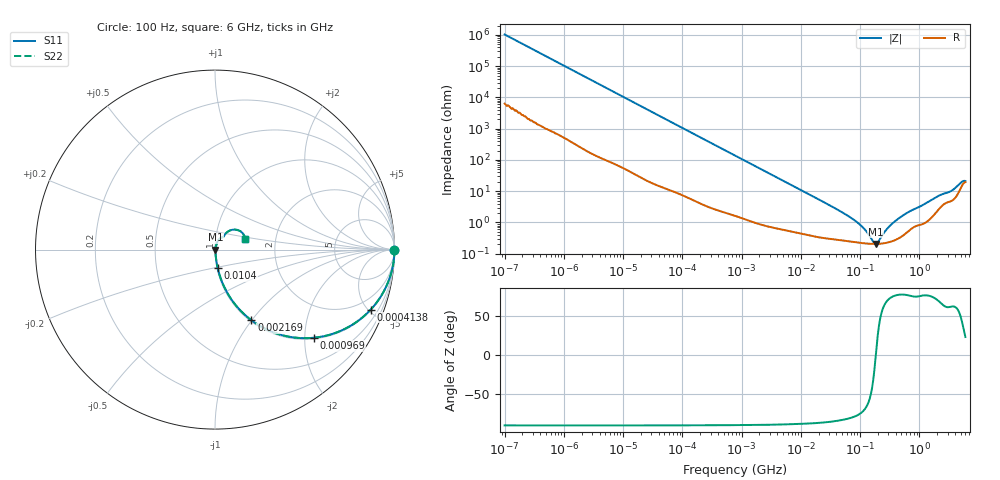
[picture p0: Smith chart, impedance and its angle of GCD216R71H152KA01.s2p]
!Murata Part Number: GCD216R71H152KA01
!These Parameters are Measured in Series Mode Connection
!Data Generated on Mar 13, 2026
!  o--ll--o
!Port1  Port2
!  o------o
!Operation Temp=25[degC], DC Bias Voltage=0[V]
!Freq. Start=100[Hz] Stop=6[GHz] 401[Steps]
# Hz S RI R 50
!Freq.(Hz) S11(Real) S11(Imag) S21(Real) S21(Imag) S12(Real) S12(Imag) S22(Real) S22(Imag)
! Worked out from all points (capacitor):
!   401 points, 100 Hz to 6 GHz, reference 50 ohm
!   read as one part in series: C = 1.53 nF near 109 Hz
!   lowest |Z| = 207 mohm at 182.6 MHz (marker M1)
!   series resonance near 184.5 MHz, so ESL is about 490 pH
!   S11 on the Smith chart (normalised r, x): 100 Hz: open; 413.8 kHz: 1.05, -5.16; 969 kHz: 1.03, -2.22; 2.169 MHz: 1.02, -0.99; 10.4 MHz: 1.01, -0.21; 6 GHz: 1.39, +0.17
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100  1 -9.63e-05  6e-07 9.63e-05  6e-07 9.63e-05  1 -9.63e-05
2008  1 -0.00192  1.24e-05 0.00192  1.24e-05 0.00192  1 -0.00192
40335  0.9983 -0.0381  0.00166 0.0381  0.00166 0.0381  0.9983 -0.0381
141303  0.9817 -0.1303  0.0183 0.1303  0.0183 0.1303  0.9817 -0.1303
413847  0.8672 -0.3348  0.1328 0.3348  0.1328 0.3348  0.8672 -0.3348
774597  0.6552 -0.4694  0.3448 0.4694  0.3448 0.4694  0.6552 -0.4694
968953  0.5504 -0.4911  0.4496 0.4911  0.4496 0.4911  0.5504 -0.4911
2169299  0.2025 -0.3934  0.7975 0.3934  0.7975 0.3934  0.2025 -0.3934
4060267  0.0716 -0.2463  0.9284 0.2463  0.9284 0.2463  0.0716 -0.2463
1.039699e7  0.0151 -0.1032  0.9849 0.1032  0.9849 0.1032  0.0151 -0.1032
1.555665e7  0.00854 -0.0696  0.9915 0.0696  0.9915 0.0696  0.00854 -0.0696
8.154455e7  0.00247 -0.0113  0.9975 0.0113  0.9975 0.0113  0.00247 -0.0113
1.166697e8  0.00219 -0.00597  0.9978 0.00597  0.9978 0.00597  0.00219 -0.00597
1.669249e8  0.00206 -0.00127  0.9979 0.00127  0.9979 0.00127  0.00206 -0.00127
1.825626e8  0.00206 -0.000133  0.9979 0.000133  0.9979 0.000133  0.00206 -0.000133
1.996653e8  0.00207 0.00101  0.9979 -0.00101  0.9979 -0.00101  0.00207 0.00101
3.124326e8  0.0024 0.00711  0.9976 -0.00711  0.9976 -0.00711  0.0024 0.00711
6.395615e8  0.00543 0.0202  0.9946 -0.0202  0.9946 -0.0202  0.00543 0.0202
2.048624e9  0.0274 0.0615  0.9726 -0.0615  0.9726 -0.0615  0.0274 0.0615
3.505958e9  0.0539 0.0822  0.9461 -0.0822  0.9461 -0.0822  0.0539 0.0822
5.016141e9  0.1253 0.1095  0.8747 -0.1095  0.8747 -0.1095  0.1253 0.1095
6e9  0.1679 0.0577  0.8321 -0.0577  0.8321 -0.0577  0.1679 0.0577
